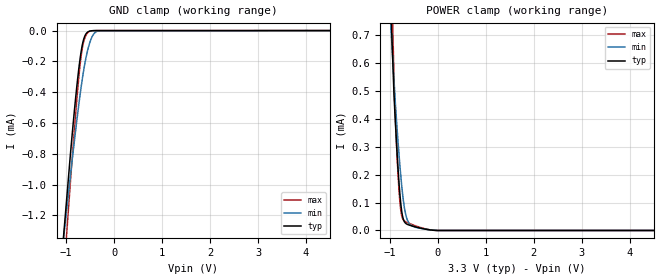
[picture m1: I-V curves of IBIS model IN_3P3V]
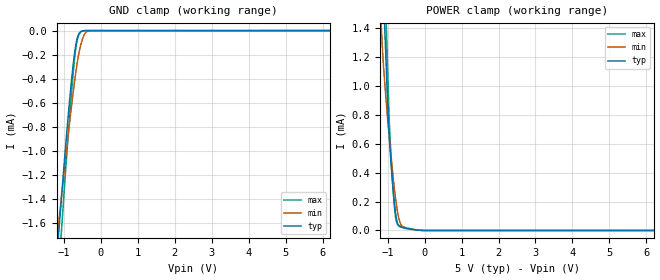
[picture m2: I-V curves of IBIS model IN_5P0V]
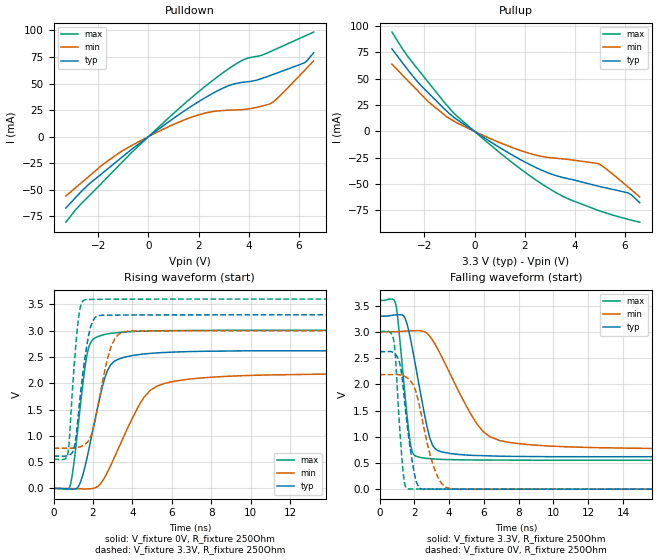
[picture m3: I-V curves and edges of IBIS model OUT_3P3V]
| Texas Instruments Incorporated
| Low-Power Single channel Digital Isolator
| Marketing part#   Voltage Range   Package-type   #pins/pkg drawing
| ISO7310C   3.0V - 5.5V   SOIC   8-pin D
[IBIS Ver]   4.1
[File name]   iso7310fc.ibs
[File Rev]   1.0
[Date]   09/30/2014
[Source]   Model built from spectre simulations at:
   Texas Instruments Incorporated.
   Analog-eLab, HPA
   12500 TI Blvd
   Dallas, TX -75243
   For Support e-mail: elab_ibis@list.ti.com
[Notes]   Revision History
   Rev 1.0: 09/30/2014
   - ccomp values are based on PVT settings:
   MIN: Low Voltage, High Temperature, Weak Process
   TYP: Nominal Voltage, Nominal Temperature, Nominal Process
   MAX: High Voltage, Low Temperature, Fast Process
   - C_comp although listed in numerical order of value are obtained from varying PVT conditions.
   For PVT conditions for each specific value, refer to the buffer description under respective [Model].
   IBIS model user is responsible for using appropriate C_comp to simulate for Signal Integrity.
[Disclaimer]  This model is designed as an aid for customers of Texas Instruments
 TI and its licensors and suppliers make no warranties, either expressed
 or implied, with respect to this  model, including the warranties of
 merchantability or fitness for a particular purpose.
 The model is provided solely on an "as is" basis. The entire risk as to
 its quality and performance is with the customer.
[Copyright] (C)Copyright 2014 Texas Instruments Incorporated.
   All rights reserved.
[Component]   ISO7310FCD
[Manufacturer]  Texas Instruments Incorporated
[Package]   |8-pin SOIC D package
|   typ   min   max
R_pkg   0.0731   0.0323   0.1488
L_pkg   2.0686n   1.4128n   3.1866n
C_pkg   0.4315p   0.3849p   0.5363p
[Pin]   signal_name   model_name   R_pin   L_pin   C_pin
1   VCC1   POWER   0.14877  3.18658n  0.42816p
2   INA   IN   0.09258  2.21690n  0.39598p
3   INB   IN   0.08330  2.07043n  0.38782p
4   GND1   GND   0.05323  1.98056n  0.41432p
5   GND2   GND   0.05034  1.89272n  0.40532p
6   OUTB   OUT   0.08318  2.07010n  0.38488p
7   OUTA   OUT   0.03229  1.41283n  0.49902p
8   VCC2   POWER   0.04142  1.71874n  0.53634p
[Model Selector] IN
IN_3P3V   3.3V Input
IN_5P0V   5.0V Input
[Model Selector] OUT
OUT_3P3V   3.3V Output
OUT_5P0V   5.0V Output
| Models and submodels in the file (4): IN_3P3V (Input), IN_5P0V (Input), OUT_3P3V (Output), OUT_5P0V (Output)
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|   Model IN_3P3V
[Model]   IN_3P3V
Model_type   Input
Vinl = .8
Vinh = 2
|   typ   min   max
|   (nom PVT)   (slow PVT)   (fast PVT)
C_comp   0.351p   0.323p   0.382p
| Where   nom PVT is  Nominal Process, 3.3V, 27C
|   Fast PVT is Strong Process, 3.6V, -40C
|   Slow PVT is Weak Process, 3.0V, 150C
[Voltage Range]   3.3   3   3.6
[Temperature Range]   27   150   -40
[Power Clamp Reference]   3.3   3   3.6
[GND Clamp Reference]   0   0   0
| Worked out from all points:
|   GND clamp passes 1 mA (typ) near -0.96 V on its own axis
|   POWER clamp passes 1 mA (typ) near -1.02 V on its own axis
[GND Clamp]
|   Voltage   I(typ)   I(min)   I(max)
-3.3V     -10.5mA    -8.177mA   -12.99mA
-1.082V   -1.445mA   -1.431mA   -1.727mA
-914.1mV  -816.9uA   -954.1uA   -998.5uA
-805.2mV  -448.8uA   -657.2uA   -556.2uA
-716.1mV  -199.7uA   -434.2uA   -244.8uA
-676.5mV  -117.1uA   -344.3uA   -142.2uA
-636.9mV  -59.87uA   -263.2uA   -75.98uA
-587.4mV  -22.32uA   -177.9uA   -31.66uA
-528mV    -5.765uA   -100.5uA   -8.109uA
-419.1mV  -436.4nA   -19.72uA   -339.2nA
-260.7mV  -145.3nA   -1.051uA   -79.88nA
6.6V      0A         0A         0A
[POWER Clamp]
|   Voltage   I(typ)   I(min)   I(max)
-3.3V     19.35mA    14.36mA    23.78mA
-1.082V   1.282mA    1.032mA    1.702mA
-914.1mV  486.5uA    539.1uA    550.7uA
-894.3mV  418uA      481uA      439.2uA
-844.8mV  262.9uA    353.4uA    248.9uA
-805.2mV  160.1uA    262.6uA    132.8uA
-775.5mV  100.8uA    201.4uA    76.11uA
-706.2mV  34.28uA    91.86uA    35.49uA
-627mV    21.23uA    34.25uA    27.78uA
-488.4mV  13.81uA    12.6uA     18.19uA
-3.3mV    4.025nA    17.39nA    2.182nA
6.6V      0A         0A         0A
|   Model IN_5P0V
[Model]   IN_5P0V
Model_type   Input
Vinl = .8
Vinh = 2
|   typ   min   max
|   (nom PVT)   (slow PVT)   (fast PVT)
C_comp   0.354p   0.325p   0.383p
| Where   nom PVT is  Nominal Process, 5.0V, 27C
|   Fast PVT is Strong Process, 5.5V, -40C
|   Slow PVT is Weak Process, 4.5V, 150C
[Voltage Range]   5   4.5   5.5
[Temperature Range]   27   150   -40
[Power Clamp Reference]   5   4.5   5.5
[GND Clamp Reference]   0   0   0
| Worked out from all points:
|   GND clamp passes 1 mA (typ) near -0.96 V on its own axis
|   POWER clamp passes 1 mA (typ) near -1.02 V on its own axis
[GND Clamp]
|   Voltage   I(typ)   I(min)   I(max)
-5V       -17.49mA   -13.39mA   -21.79mA
-1.265V   -2.166mA   -1.968mA   -2.56mA
-1.13V    -1.641mA   -1.569mA   -1.954mA
-1.115V   -1.583mA   -1.526mA   -1.887mA
-1.055V   -1.349mA   -1.352mA   -1.617mA
-875mV    -679.6uA   -844.2uA   -834.7uA
-740mV    -259.5uA   -491.7uA   -320.4uA
-650mV    -75.81uA   -288.9uA   -93.96uA
-515mV    -4.2uA     -86.9uA    -5.717uA
-410mV    -367.7nA   -16.42uA   -267.5nA
-290mV    -148.8nA   -1.483uA   -81.78nA
10V       0A         0A         0A
[POWER Clamp]
|   Voltage   I(typ)   I(min)   I(max)
-5V       33.7mA     25.28mA    41.1mA
-1.265V   2.636mA    1.846mA    3.37mA
-1.13V    1.74mA     1.206mA    2.217mA
-1.085V   1.441mA    1.042mA    1.833mA
-1.04V    1.143mA    894.1uA    1.449mA
-1.025V   1.043mA    847.5uA    1.321mA
-980mV    744.9uA    713.8uA    937.1uA
-950mV    621.2uA    628.7uA    718.6uA
-845mV    264uA      354.7uA    250.1uA
-770mV    92.28uA    191.7uA    69.37uA
-650mV    23.46uA    45.43uA    29.88uA
10V       0A         0A         0A
|   Model OUT_3P3V
[Model]   OUT_3P3V
Model_type   Output
Polarity   Non-Inverting
Vmeas = 1.65
Vref = 3.3
Cref = 15pF
Rref = 250
|   typ   min   max
|   (fast PVT)   (slow PVT)   (nom PVT)
C_comp   0.728p   0.678p   0.736p
|C_comp (ON state)   0.797p   0.677p   0.792p
|C_comp (OFF state)   0.728p   0.678p   0.736p
| Where   nom PVT is  Nominal Process, 3.3V, 27C
|   Fast PVT is Strong Process, 3.6V, -40C
|   Slow PVT is Weak Process, 3.0V, 150C
[Voltage Range]   3.3   3   3.6
[Temperature Range]   27   150   -40
[Pullup Reference]   3.3   3   3.6
[Pulldown Reference]   0   0   0
[Power Clamp Reference]   3.3   3   3.6
[GND Clamp Reference]   0   0   0
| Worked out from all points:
|   slope of the pulldown table from 0 to 0.495 V, typ, clamps not added: 57 ohm
|   slope of the pullup table from 0 to 0.495 V, typ, clamps not added: 64.2 ohm
|   falling waveform, V_fixture 3.3V, R_fixture 250Ohm: 20-80 % time 916ps typ, 2.14ns min, 533ps max; typ from 3.3 V to 0.619 V
|   rising waveform, V_fixture 0V, R_fixture 250Ohm: 20-80 % time 931ps typ, 1.72ns min, 562ps max; typ from 0 V to 2.62 V
|   rising waveform, V_fixture 3.3V, R_fixture 250Ohm: 20-80 % time 518ps typ, 737ps min, 353ps max; typ from 0.615 V to 3.3 V
|   falling waveform, V_fixture 0V, R_fixture 250Ohm: 20-80 % time 578ps typ, 919ps min, 346ps max; typ from 2.62 V to 0 V
[Pulldown]
|   Voltage   I(typ)   I(min)   I(max)
-3.3V     -67.22mA   -55.92mA   -80.59mA
-2.389V   -44.97mA   -37.58mA   -56.09mA
-1.825V   -34.09mA   -26.21mA   -42.69mA
-696.3mV  -12.36mA   -8.646mA   -15.48mA
1.264V    21.55mA    14.15mA    27.39mA
2.65V     41.81mA    23.88mA    54.48mA
3.204V    47.99mA    24.92mA    63.99mA
3.729V    51.07mA    25.44mA    71.61mA
4.333V    53.29mA    27.64mA    75.66mA
4.897V    57.9mA     31.35mA    80.38mA
6.224V    69.48mA    62.11mA    94.52mA
6.6V      79.07mA    71.42mA    98.5mA
[Pullup]
|   Voltage   I(typ)   I(min)   I(max)
-3.3V     78.34mA    63.86mA    94.3mA
-2.686V   59.07mA    48.62mA    71.72mA
-2.32V    48.24mA    39.71mA    60.7mA
-1.825V   36.03mA    27.72mA    45.95mA
-1.099V   18.97mA    13.68mA    24.69mA
-696.3mV  11.13mA    8.021mA    14.38mA
1.68V     -24.78mA   -16.86mA   -32.82mA
2.511V    -35.01mA   -22.84mA   -47.11mA
3.343V    -42.61mA   -25.69mA   -59.28mA
4.947V    -52.03mA   -30.8mA    -75.05mA
6.125V    -58.4mA    -52.6mA    -83.42mA
6.6V      -67.78mA   -62.18mA   -86.22mA
[Ramp]
R_load = 250
|   typ   min   max
dV/dt_r   1.57011/9.31334e-10   1.30951/1.7182e-09   1.80445/5.62179e-10
dV/dt_f   1.60858/9.15648e-10   1.33827/2.13619e-09   1.8288/5.32895e-10
[Falling Waveform]
V_fixture = 3.3V
V_fixture_min = 3V
V_fixture_max = 3.6V
R_fixture = 250Ohm
C_fixture = 0F
|   Time   V(typ)   V(min)   V(max)
0s        3.3V       3V         3.6V
926.7ps   3.323V     3.003V     3.535V
1.391ns   3.302V     3.013V     2.046V
1.701ns   2.986V     3.018V     1.037V
2.122ns   2.256V     3.023V     625.9mV
2.72ns    1.202V     2.975V     586.9mV
3.195ns   771.1mV    2.761V     573.9mV
5.606ns   641.9mV    1.24V      556.8mV
6.908ns   629.1mV    927.6mV    554.9mV
19.9ns    619mV      769.6mV    552mV
[Rising Waveform]
V_fixture = 0V
V_fixture_min = 0V
V_fixture_max = 0V
R_fixture = 250Ohm
C_fixture = 0F
|   Time   V(typ)   V(min)   V(max)
0s        649.2pV    4.074nV    572.1pV
854.3ps   -10.96mV   -1.995mV   72.08mV
1.281ns   49.65mV    -6.905mV   1.3V
1.701ns   588.6mV    -8.959mV   2.553V
2.217ns   1.514V     31.88mV    2.883V
2.72ns    2.232V     302.2mV    2.936V
3.041ns   2.406V     554.2mV    2.954V
4.589ns   2.556V     1.736V     2.99V
5.606ns   2.584V     1.995V     2.999V
19.9ns    2.617V     2.183V     3.007V
[Rising Waveform]
V_fixture = 3.3V
V_fixture_min = 3V
V_fixture_max = 3.6V
R_fixture = 250Ohm
C_fixture = 0F
|   Time   V(typ)   V(min)   V(max)
0s        614.5mV    765mV      551.6mV
743.1ps   625.3mV    764.6mV    691.4mV
1.08ns    826mV      770.3mV    2.499V
1.218ns   1.252V     778.5mV    3.081V
1.571ns   2.429V     832.8mV    3.584V
1.876ns   3.071V     985.5mV    3.592V
2.107ns   3.25V      1.285V     3.594V
2.927ns   3.294V     2.707V     3.597V
3.58ns    3.296V     2.978V     3.598V
19.9ns    3.3V       3V         3.6V
[Falling Waveform]
|Gnd
V_fixture = 0V
V_fixture_min = 0V
V_fixture_max = 0V
R_fixture = 250Ohm
C_fixture = 0F
|   Time   V(typ)   V(min)   V(max)
0s        2.622V     2.184V     3.008V
815.5ps   2.601V     2.185V     2.839V
1.291ns   2.129V     2.171V     554.4mV
1.447ns   1.65V      2.152V     98.37mV
1.571ns   1.269V     2.127V     11.61mV
1.98ns    330.9mV    1.954V     2.742mV
2.22ns    54.41mV    1.701V     2.389mV
3.1ns     2.141mV    439.6mV    1.097mV
3.799ns   1.619mV    39.07mV    784.2uV
19.9ns    121uV      48.77uV    33.25uV
